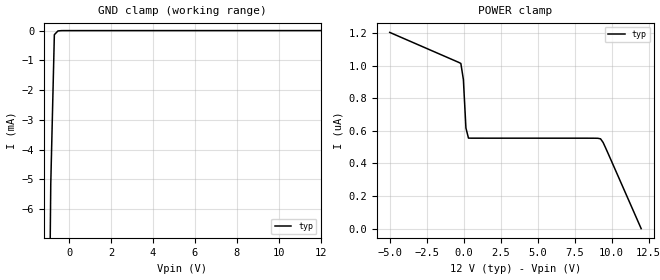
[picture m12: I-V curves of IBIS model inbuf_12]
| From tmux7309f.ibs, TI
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| inbuf_12
[Model]   inbuf_12
Model_type   Input
Vinl = 0.8
Vinh = 1.3
|   typ   min   max
C_comp   6.362683e-13   NA   NA
[Voltage Range]   12   NA   NA
[Temperature Range]   27   NA   NA
[Power Clamp Reference]   12   NA   NA
[GND Clamp Reference]   0   NA   NA
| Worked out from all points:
|   GND clamp passes 1 mA (typ) near -0.74 V on its own axis
[GND Clamp]
|   Voltage   I(typ)   I(min)   I(max)
-5V       -369.9mA   NA         NA
-1.051V   -17.4mA    NA         NA
-878.8mV  -5.168mA   NA         NA
-707.1mV  -136.9uA   NA         NA
-535.4mV  -10.86uA   NA         NA
12V       881.5nA    NA         NA
[POWER Clamp]
|   Voltage   I(typ)   I(min)   I(max)
-5V       1.203uA    NA         NA
-191.9mV  1.013uA    NA         NA
-20.2mV   914.5nA    NA         NA
151.5mV   617.2nA    NA         NA
323.2mV   555nA      NA         NA
9.253V    550.5nA    NA         NA
9.424V    528.7nA    NA         NA
9.596V    495nA      NA         NA
12V       -76.65pA   NA         NA
